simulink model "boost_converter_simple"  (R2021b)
settings: Solver=ode23tb  StartTime=0.0  StopTime=20  MaxStep=0.01  RelTol=1e-3  EnableMultiTasking=on
undefined symbols (not defined in the file or in its folder): BLOCKS, example, Frequency, Junction, Limited, n, Parallel, Series, SIMBUS, SIMBUS_BONDGRAPHS
libraries: lib_connector x4, lib_select_power_variable x4, lib_zero_junction x2, lib_generic_resistance x2, lib_one_junction x1, lib_generic_capacitance x1, lib_generic_inertance x1, lib_modulated_transformer x1, lib_simbus_extras x1, lib_effort_source x1

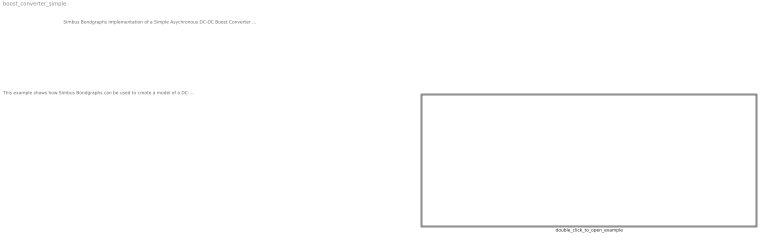
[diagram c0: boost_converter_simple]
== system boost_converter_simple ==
  note: Simbus Bondgraphs Implementation of a Simple Asychronous DC-DC Boost Converter v3
  note: This example shows how Simbus Bondgraphs can be used to create a model of a DC-DC boost (voltage step-up) converter. This particular boost converter description is one of the simplest possible and consists of only four components: an inductor, a diode, a semiconductor switch (such as a MOSFET or an IGBT ), and an output capacitor. This kind of converter uses a single switch and is known as an Asynchronous Converter. A Sychronous Converter is one where the diode is replaced by another semiconductor switch. A voltage source is attached to the input and a load impedance is attached to the output. The should be provided at the A-side and B-side of the converter block respectively. The formulas used by the block to size the internal components assume that the boost converter operates in continuous conduction mode. Good starting points to understand the operation of this boost converter can be found in this article and in this video . The boost converter is implemented as a reusable block. Make sure to distribute blk_boost_converter_simple.p and blk_boost_converter_simple.m if you use and share this block in your own models. Copyright and licensing information for the circuit image is available here .
  double_click_to_open_example : Subsystem

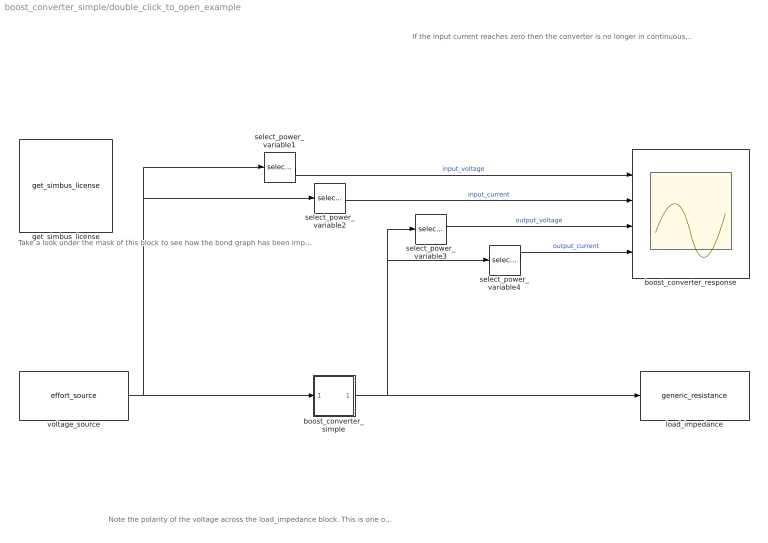
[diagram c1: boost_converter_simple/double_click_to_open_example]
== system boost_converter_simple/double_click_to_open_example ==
  note: Note the polarity of the voltage across the load_impedance block. This is one of the simplest converter topologies and inverts the voltage polarity with respect to its input. Take a look at SEPIC , zeta converter , or a two-switch buck-boost converter if you need noninverting operation.
  note: Take a look under the mask of this block to see how the bond graph has been implemented and how it relates to the circuit at the top level of this model.
  note: If the input current reaches zero then the converter is no longer in continuous conduction mode.
  boost_converter_response : Scope  NumInputPorts=4
  boost_converter_simple : Subsystem  mask(Simple DC-DC Boost Converter){simbus_vendor=SIMBUS, simbus_toolbox=SIMBUS_BONDGRAPHS, simbus_component=BLOCKS, simbus_class=example.converter.boost_converter_simple, msk_V_in=12, msk_V_out=36, msk_Z_out_min=12, msk_inductor_I_ripple_percent=20, msk_capacitance_V_ripple_percent=4, msk_f_switch=100000}
      mask prompts: simbus_vendor "Vendor:"; simbus_toolbox "Toolbox:"; simbus_component "Component:"; simbus_class "Class:"; msk_V_in "Input Voltage (V):"; msk_V_out "Desired Output Voltage (V):"; msk_Z_out_min "Minimum Output Impedance (ohm):"; msk_inductor_I_ripple_percent "Maximum Inductor Current Ripple (% of average):"; msk_capacitance_V_ripple_percent "Maximum Capacitance Voltage Ripple (% of average):"; msk_f_switch "Switching Frequency (Hz):"
      mask help: This block demonstrates the fundamental operation of a DC-DC boost (step-up) converter using bond graphs. Boost converters use two switches to alternately connect the internal inductor to ground (0 V) or to an output capacitor that integrates the current to create the output voltage. The switch that connects the inductor to ground is usually a switching device such as a MOSFET or IGBT. This block uses a modulated transformer junction to implement this switch. The second switch may also be implemented by a MOSFET or IGBT but in this case is implemented using a diode. This diode is described as 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
      mask init:
      | blk_params = blk_boost_converter_simple(gcb);
  get_simbus_license : lib_simbus_extras/get_simbus_license  simbus_vendor=SIMBUS  simbus_toolbox=SIMBUS_CORE  simbus_component=BLOCKS  simbus_class=core.utils.get_simbus_license
  load_impedance : lib_generic_resistance/generic_resistance  simbus_vendor=SIMBUS  simbus_toolbox=SIMBUS_BONDGRAPHS  simbus_component=BLOCKS  simbus_class=bond.1_port.generic_resistance  msk_physical_domain=Generic  msk_connection_point=B  msk_computed_pv=Flow  msk_lock_causality=off  msk_computation_method=Linear Relation  msk_resistance=12  msk_effort_table=[0 0; 1 1]  msk_effort_interp_method=Linear point-slope  msk_effort_extrap_method=Linear  msk_flow_table=[0 0; 1 1]  msk_flow_interp_method=Linear point-slope  msk_flow_extrap_method=Linear  msk_index_search_method=Linear search  msk_index_search_using_previous=on  msk_effort_expr=u  msk_flow_expr=u*sin(u)  msk_icon_type=Default  msk_icon_source=Generic\nResistance
  select_power_variable1 : lib_select_power_variable/select_power_variable  simbus_vendor=SIMBUS  simbus_toolbox=SIMBUS_BONDGRAPHS  simbus_component=BLOCKS  simbus_class=measurement.select_power_variable  msk_pv_name=Effort  msk_bond_idx=1  msk_multibond_connected=logical(false)
  select_power_variable2 : lib_select_power_variable/select_power_variable  simbus_vendor=SIMBUS  simbus_toolbox=SIMBUS_BONDGRAPHS  simbus_component=BLOCKS  simbus_class=measurement.select_power_variable  msk_pv_name=Flow  msk_bond_idx=1  msk_multibond_connected=logical(false)
  select_power_variable3 : lib_select_power_variable/select_power_variable  simbus_vendor=SIMBUS  simbus_toolbox=SIMBUS_BONDGRAPHS  simbus_component=BLOCKS  simbus_class=measurement.select_power_variable  msk_pv_name=Effort  msk_bond_idx=1  msk_multibond_connected=logical(false)
  select_power_variable4 : lib_select_power_variable/select_power_variable  simbus_vendor=SIMBUS  simbus_toolbox=SIMBUS_BONDGRAPHS  simbus_component=BLOCKS  simbus_class=measurement.select_power_variable  msk_pv_name=Flow  msk_bond_idx=1  msk_multibond_connected=logical(false)
  voltage_source : lib_effort_source/effort_source  simbus_vendor=SIMBUS  simbus_toolbox=SIMBUS_BONDGRAPHS  simbus_component=BLOCKS  simbus_class=bond.1_port.effort_source  msk_physical_domain=Generic  msk_connection_point=A  msk_power_direction=B => A  msk_effort_value=12  msk_icon_type=Default  msk_icon_source=Effort\nSource
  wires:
  boost_converter_simple/1(B) -> select_power_variable4/1, select_power_variable3/1, load_impedance/1
  voltage_source/1 -> boost_converter_simple/1(A), select_power_variable1/1, select_power_variable2/1
  select_power_variable1/1 -> boost_converter_response/1  "input_voltage"
  select_power_variable2/1 -> boost_converter_response/2  "input_current"
  select_power_variable3/1 -> boost_converter_response/3  "output_voltage"
  select_power_variable4/1 -> boost_converter_response/4  "output_current"

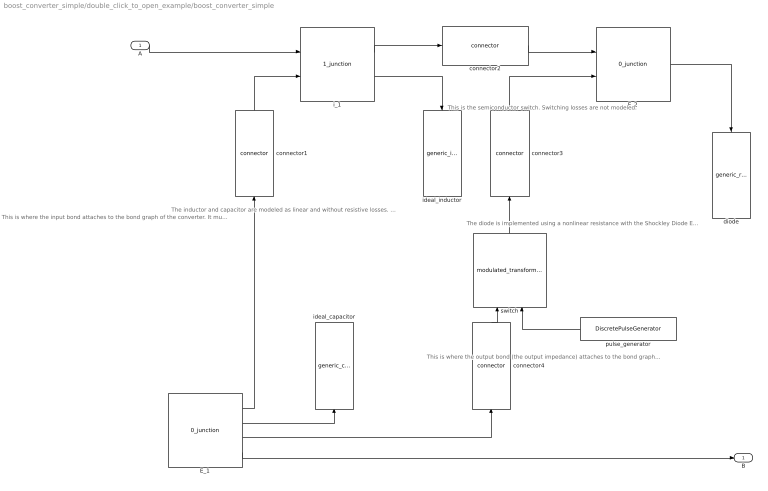
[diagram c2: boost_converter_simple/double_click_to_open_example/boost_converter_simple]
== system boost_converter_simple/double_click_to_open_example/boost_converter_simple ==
  note: This is where the input bond attaches to the bond graph of the converter. It must provide effort (voltage) here.
  note: This is the semiconductor switch. Switching losses are not modeled.
  note: The diode is implemented using a nonlinear resistance with the Shockley Diode Equation as the user-defined function.
  note: This is where the output bond (the output impedance) attaches to the bond graph of the converter. It must provide flow (current) here.
  note: The inductor and capacitor are modeled as linear and without resistive losses. Thermal behavior is not modeled.
  A : Inport
  E_1 : lib_zero_junction/0_junction  simbus_vendor=SIMBUS  simbus_toolbox=SIMBUS_BONDGRAPHS  simbus_component=BLOCKS  simbus_class=bond.3_port.0_junction  msk_physical_domain=Generic  msk_num_a_side_ports=0  msk_num_b_side_ports=4  msk_icon_type=Default  msk_icon_source=0-Junction\n(Parallel Junction)
  E_2 : lib_zero_junction/0_junction  simbus_vendor=SIMBUS  simbus_toolbox=SIMBUS_BONDGRAPHS  simbus_component=BLOCKS  simbus_class=bond.3_port.0_junction  msk_physical_domain=Generic  msk_num_a_side_ports=2  msk_num_b_side_ports=1  msk_icon_type=Default  msk_icon_source=0-Junction\n(Parallel Junction)
  connector1 : lib_connector/connector  simbus_vendor=SIMBUS  simbus_toolbox=SIMBUS_BONDGRAPHS  simbus_component=BLOCKS  simbus_class=bond.connector.connector  msk_physical_domain=Generic  msk_power_direction=B => A  msk_causal_stroke_location=A  msk_lock_causality=on  msk_icon_type=Default  msk_icon_source=Connector
  connector2 : lib_connector/connector  simbus_vendor=SIMBUS  simbus_toolbox=SIMBUS_BONDGRAPHS  simbus_component=BLOCKS  simbus_class=bond.connector.connector  msk_physical_domain=Generic  msk_power_direction=B => A  msk_causal_stroke_location=B  msk_lock_causality=on  msk_icon_type=Default  msk_icon_source=Connector
  connector3 : lib_connector/connector  simbus_vendor=SIMBUS  simbus_toolbox=SIMBUS_BONDGRAPHS  simbus_component=BLOCKS  simbus_class=bond.connector.connector  msk_physical_domain=Generic  msk_power_direction=B <= A  msk_causal_stroke_location=A  msk_lock_causality=on  msk_icon_type=Default  msk_icon_source=Connector
  connector4 : lib_connector/connector  simbus_vendor=SIMBUS  simbus_toolbox=SIMBUS_BONDGRAPHS  simbus_component=BLOCKS  simbus_class=bond.connector.connector  msk_physical_domain=Generic  msk_power_direction=B <= A  msk_causal_stroke_location=A  msk_lock_causality=on  msk_icon_type=Default  msk_icon_source=Connector
  diode : lib_generic_resistance/generic_resistance  simbus_vendor=SIMBUS  simbus_toolbox=SIMBUS_BONDGRAPHS  simbus_component=BLOCKS  simbus_class=bond.1_port.generic_resistance  msk_physical_domain=Generic  msk_connection_point=B  msk_computed_pv=Flow  msk_lock_causality=on  msk_computation_method=User-Defined Function  msk_resistance=2  msk_effort_table=[0 0; 1 1]  msk_effort_interp_method=Linear point-slope  msk_effort_extrap_method=Linear  msk_flow_table=[0 0; 1 1]  msk_flow_interp_method=Linear point-slope  msk_flow_extrap_method=Linear  msk_index_search_method=Linear search  msk_index_search_using_previous=on  msk_effort_expr=u  msk_flow_expr=1e-12*(exp(19.2308*u)-1)  msk_icon_type=Default  msk_icon_source=Generic\nResistance
  i_1 : lib_one_junction/1_junction  simbus_vendor=SIMBUS  simbus_toolbox=SIMBUS_BONDGRAPHS  simbus_component=BLOCKS  simbus_class=bond.3_port.1_junction  msk_physical_domain=Generic  msk_num_a_side_ports=2  msk_num_b_side_ports=2  msk_icon_type=Default  msk_icon_source=1-Junction\n(Series Junction)
  ideal_capacitor : lib_generic_capacitance/generic_capacitance  simbus_vendor=SIMBUS  simbus_toolbox=SIMBUS_BONDGRAPHS  simbus_component=BLOCKS  simbus_class=bond.1_port.generic_capacitance  msk_physical_domain=Generic  msk_connection_point=B  msk_computed_pv=Effort  msk_lock_causality=on  msk_computation_method=Linear Relation  msk_capacitance=blk_params.C  msk_effort_table=[0 0; 1 1]  msk_effort_interp_method=Linear point-slope  msk_effort_extrap_method=Linear  msk_displacement_table=[0 0; 1 1]  msk_displacement_interp_method=Linear point-slope  msk_displacement_extrap_method=Linear  msk_index_search_method=Binary search  msk_index_search_using_previous=on  msk_effort_expr=u  msk_displacement_expr=u  msk_int_tol=auto  msk_time_derivative_type=Simple  msk_highest_freq_hz=10  msk_freq_break_factor=2  msk_roll_off_factor=3  msk_q0=0  msk_f0=0  msk_icon_type=Default  msk_icon_source=Generic\nCapacitance
  ideal_inductor : lib_generic_inertance/generic_inertance  simbus_vendor=SIMBUS  simbus_toolbox=SIMBUS_BONDGRAPHS  simbus_component=BLOCKS  simbus_class=bond.1_port.generic_inertance  msk_physical_domain=Generic  msk_connection_point=B  msk_computed_pv=Flow  msk_lock_causality=on  msk_computation_method=Linear Relation  msk_inertance=blk_params.L  msk_momentum_table=[0 0; 1 1]  msk_momentum_interp_method=Linear point-slope  msk_momentum_extrap_method=Linear  msk_flow_table=[0 0; 1 1]  msk_flow_interp_method=Linear point-slope  msk_flow_extrap_method=Linear  msk_index_search_method=Binary search  msk_index_search_using_previous=on  msk_momentum_expr=(u>0.25)*u^(0.5)+(u<=0.25)*u^(1/3)  msk_flow_expr=u*sin(u)  msk_int_tol=auto  msk_time_derivative_type=Frequency-Limited  msk_highest_freq_hz=10  msk_freq_break_factor=2  msk_roll_off_factor=3  msk_p0=0  msk_e0=3  msk_icon_type=Default  msk_icon_source=Generic\nInertance
  pulse_generator : DiscretePulseGenerator  PulseType=Time based  Period=blk_params.T_switch  PulseWidth=blk_params.duty_cycle_percent
  switch : lib_modulated_transformer/modulated_transformer  simbus_vendor=SIMBUS  simbus_toolbox=SIMBUS_BONDGRAPHS  simbus_component=BLOCKS  simbus_class=bond.2_port.modulated_transformer  msk_a_side_physical_domain=Generic  msk_b_side_physical_domain=Generic  msk_icon_type=Default  msk_icon_source=Modulated\nTransformer\nJunction
  B : Outport
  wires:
  E_1/3 -> connector4/1
  E_1/2 -> ideal_capacitor/1
  i_1/2 -> ideal_inductor/1
  A/1 -> i_1/1
  E_1/1 -> connector1/1
  connector3/1 -> E_2/2
  connector1/1 -> i_1/2
  E_1/4 -> B/1
  switch/1 -> connector3/1
  E_2/1 -> diode/1
  connector4/1 -> switch/1
  connector2/1 -> E_2/1
  i_1/1 -> connector2/1
  pulse_generator/1 -> switch/2
